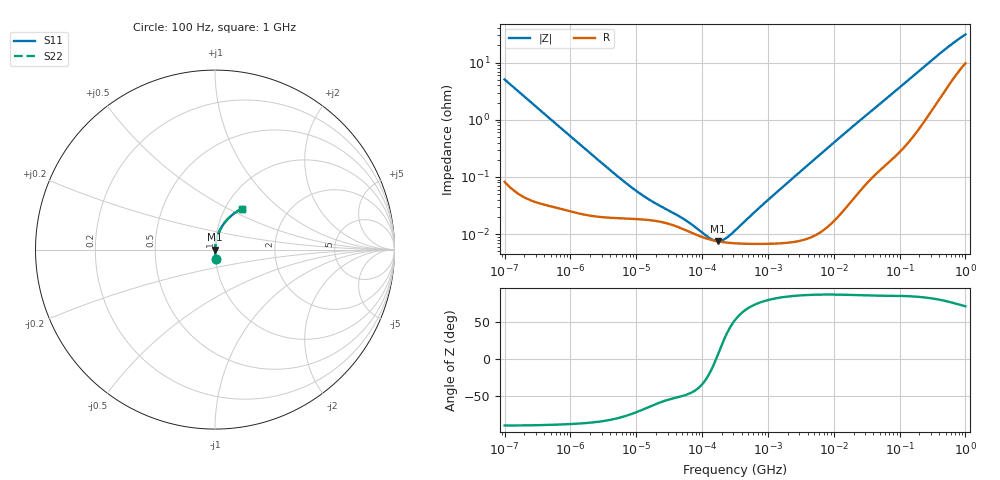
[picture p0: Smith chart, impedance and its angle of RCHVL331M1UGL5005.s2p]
! RCHVL331M1UGL5005  S-PARAMETER MODEL  (AEC-Q200 qualified)
! Model Generated by ELNA Corporation (http://www.ty-top.com)
! Version 1.0
! ELNA Control No. 231122
! Copyright (c) 2023 ELNA CO.,LTD. All Rights Reserved.
! Products Name : CONDUCTIVE POLYMER HYBRID ALUMINUM ELECTROLYTIC CAPACITORS
! Characteristics :
!  Capacitance  :  330uF  ,  Rated voltage  :  50V
!  Operating Temp. Range  :  -55 to +125 degC  ,  Endurance  :  84000hr at 125 degC
!  Dimension D  :  12.5mm  ,  Dimension L  :  13.5mm
! Frequency Range : 100Hz - 1GHz
! External Node Assignments :
!  1  o---| |---o  2
# MHz S RI R 50
!Freq[MHz].  S11 Real  S11 Imag  S21 Real  S21 Imag  S12 Real  S12 Imag  S22 Real  S22 Imag
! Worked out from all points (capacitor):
!   401 points, 100 Hz to 1 GHz, reference 50 ohm
!   read as one part in series: C = 313 uF near 108 Hz
!   lowest |Z| = 7.52 mohm at 172.8 kHz (marker M1)
!   series resonance near 162.2 kHz, so ESL is about 3.1 nH
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0.0001  0.00339 -0.0506  0.9966 0.0506  0.9966 0.0506  0.00339 -0.0506
0.000113  0.00273 -0.0449  0.9973 0.0449  0.9973 0.0449  0.00273 -0.0449
0.000309  0.000627 -0.0165  0.9994 0.0165  0.9994 0.0165  0.000627 -0.0165
0.001488  0.000236 -0.00347  0.9998 0.00347  0.9998 0.00347  0.000236 -0.00347
0.004241  0.000194 -0.00123  0.9998 0.00123  0.9998 0.00123  0.000194 -0.00123
0.008082  0.000186 -0.000659  0.9998 0.000659  0.9998 0.000659  0.000186 -0.000659
0.013646  0.000179 -0.000407  0.9998 0.000407  0.9998 0.000407  0.000179 -0.000407
0.022131  0.000166 -0.000272  0.9998 0.000272  0.9998 0.000272  0.000166 -0.000272
0.051582  0.000122 -0.00014  0.9999 0.00014  0.9999 0.00014  0.000122 -0.00014
0.106537  8.64e-05 -5.14e-05  0.9999 5.14e-05  0.9999 5.14e-05  8.64e-05 -5.14e-05
0.172783  7.48e-05 7.9e-06  0.9999 -7.9e-06  0.9999 -7.9e-06  7.48e-05 7.9e-06
0.258523  7.02e-05 6.16e-05  0.9999 -6.16e-05  0.9999 -6.16e-05  7.02e-05 6.16e-05
0.280221  6.96e-05 7.34e-05  0.9999 -7.34e-05  0.9999 -7.34e-05  6.96e-05 7.34e-05
0.316228  6.9e-05 9.21e-05  0.9999 -9.21e-05  0.9999 -9.21e-05  6.9e-05 9.21e-05
0.865964  6.74e-05 0.000333  0.9999 -0.000333  0.9999 -0.000333  6.74e-05 0.000333
4.704354  9.31e-05 0.00187  0.9999 -0.00187  0.9999 -0.00187  9.31e-05 0.00187
17.78279  0.000403 0.00699  0.9996 -0.00699  0.9996 -0.00699  0.000403 0.00699
69.9842  0.00251 0.0259  0.9975 -0.0259  0.9975 -0.0259  0.00251 0.0259
169.8244  0.00917 0.0607  0.9908 -0.0607  0.9908 -0.0607  0.00917 0.0607
350.7519  0.0321 0.1175  0.9679 -0.1175  0.9679 -0.1175  0.0321 0.1175
641.9482  0.0852 0.1838  0.9148 -0.1838  0.9148 -0.1838  0.0852 0.1838
1000  0.1505 0.2289  0.8495 -0.2289  0.8495 -0.2289  0.1505 0.2289
